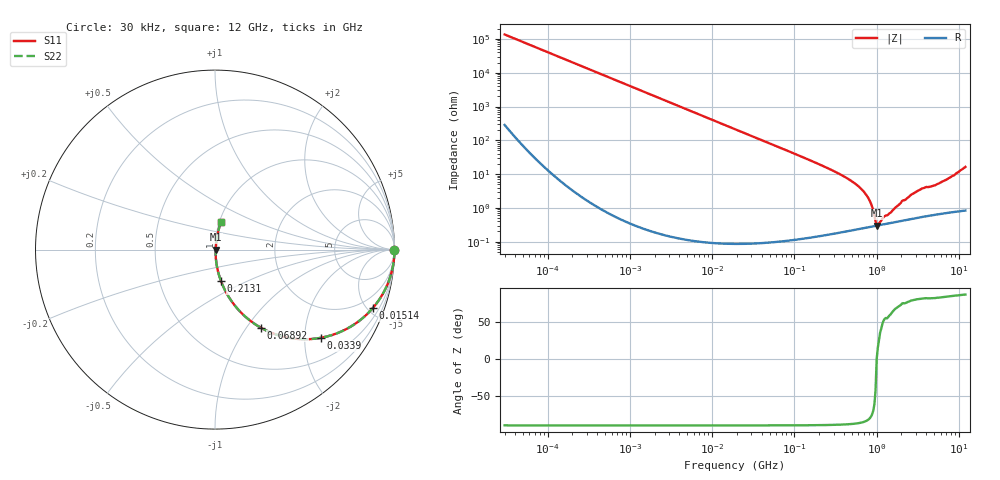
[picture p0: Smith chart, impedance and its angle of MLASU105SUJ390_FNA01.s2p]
! MLASU105SUJ390_FNA01  S-PARAMETER MODEL  ( General Type )
! Model Generated by TAIYO YUDEN Corporation (http://www.ty-top.com)
! Version 4.0
! TAIYO YUDEN Control No. 120810
! Copyright(c) 2003 TAIYO YUDEN CO.,LTD. All Rights Reserved.
! Product Description (link to TY-COMPAS)
! https://ds.yuden.co.jp/TYCOMPAS/or/detail?pn=MLASU105SUJ390JFNA01&u=M
! Products Name : Multilayer Ceramic Capacitors
! Characteristics :
!  Capacitance : 39 pF , Rated Voltage : 50V , TCC : UJ / U2J
!  Case Size : 1.0 x 0.5 / 0.039 x 0.02 [mm/inch] , Thickness : 0.5 / 0.02 [mm/inch]
!  (Conditions: Temperature = 25 degC , DC Bias Current/Voltage = 0A / 0V)
! External Node Assignments :
!  1  o---| |---o  2
! GND o---------o GND
! Frequency Range : 0.03MHz  -  12000MHz  [ 401 STEP ]
# MHz S RI R 50
! Freq[MHz].  S11 Real  S11 Imag  S21 Real  S21 Imag  S12 Real  S12 Imag  S22 Real  S22 Imag
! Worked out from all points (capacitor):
!   401 points, 30 kHz to 12 GHz, reference 50 ohm
!   read as one part in series: C = 39.1 pF near 32 kHz
!   lowest |Z| = 299 mohm at 1.002 GHz (marker M1)
!   series resonance near 1.002 GHz, so ESL is about 650 pH
!   S11 on the Smith chart (normalised r, x): 30 kHz: open; 15.14 MHz: 1.00, -5.38; 33.9 MHz: 1.00, -2.40; 68.92 MHz: 1.00, -1.18; 213.1 MHz: 1.00, -0.36; 12 GHz: 1.02, +0.33
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0.03  1 -0.000737  2.09e-06 0.000737  2.09e-06 0.000737  1 -0.000737
0.260295  1 -0.00639  4.17e-05 0.00639  4.17e-05 0.00639  1 -0.00639
2.258455  0.9969 -0.0553  0.00307 0.0553  0.00307 0.0553  0.9969 -0.0553
6.13721  0.9777 -0.1474  0.0223 0.1474  0.0223 0.1474  0.9777 -0.1474
15.13963  0.8783 -0.3267  0.1217 0.3267  0.1217 0.3267  0.8783 -0.3267
18.97367  0.8213 -0.3829  0.1787 0.3829  0.1787 0.3829  0.8213 -0.3829
33.90345  0.5898 -0.4915  0.4102 0.4915  0.4102 0.4915  0.5898 -0.4915
68.9219  0.2572 -0.4362  0.7428 0.4362  0.7428 0.4362  0.2572 -0.4362
164.6252  0.0558 -0.2269  0.9442 0.2269  0.9442 0.2269  0.0558 -0.2269
213.0775  0.0335 -0.176  0.9665 0.176  0.9665 0.176  0.0335 -0.176
433.1624  0.00778 -0.0757  0.9922 0.0757  0.9922 0.0757  0.00778 -0.0757
658.7456  0.00367 -0.0349  0.9963 0.0349  0.9963 0.0349  0.00367 -0.0349
825.5698  0.00297 -0.0158  0.997 0.0158  0.997 0.0158  0.00297 -0.0158
1001.808  0.00298 5.47e-06  0.997 -5.47e-06  0.997 -5.47e-06  0.00298 5.47e-06
1068.55  0.00308 0.00147  0.9969 -0.00147  0.9969 -0.00147  0.00308 0.00147
1215.67  0.00329 0.00415  0.9967 -0.00415  0.9967 -0.00415  0.00329 0.00415
1428.372  0.00356 0.00579  0.9964 -0.00579  0.9964 -0.00579  0.00356 0.00579
1971.936  0.00428 0.0134  0.9957 -0.0134  0.9957 -0.0134  0.00428 0.0134
2811.574  0.00551 0.0262  0.9945 -0.0262  0.9945 -0.0262  0.00551 0.0262
3758.338  0.00691 0.038  0.9931 -0.038  0.9931 -0.038  0.00691 0.038
5534.236  0.00888 0.0498  0.9911 -0.0498  0.9911 -0.0498  0.00888 0.0498
12000  0.0335 0.1563  0.9665 -0.1563  0.9665 -0.1563  0.0335 0.1563
